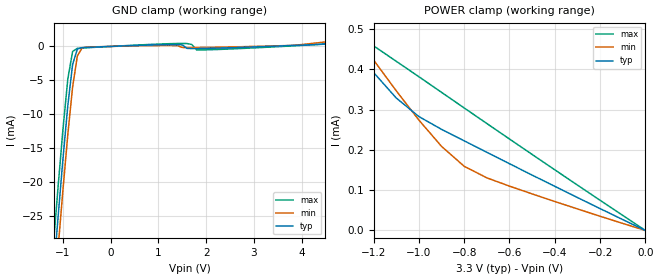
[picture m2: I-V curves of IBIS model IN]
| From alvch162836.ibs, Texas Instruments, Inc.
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|   Model ALVCH162836_IN
[Model]   IN
Model_type   Input
Polarity   Non-Inverting
Vinl = 0.8V
Vinh = 2.0V
|Variable   typ   min   max
C_comp   6pF   NA   NA
[Voltage Range]   3.3   3.0   3.6
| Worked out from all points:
|   GND clamp passes 1 mA (typ) near -0.73 V on its own axis
|   POWER clamp passes 1 mA (typ) near -1.97 V on its own axis
[POWER_Clamp]   | Note: Vtable = Vcc - Voutput
|   Voltage   I(typ)   I(min)   I(max)
-3.3V     2.121mA    2.168mA    2.076mA
-1.4V     540.7uA    581.6uA    541.7uA
-1.3V     464.2uA    501.6uA    497.2uA
-1.2V     392uA      423uA      458.1uA
-1.1V     328.8uA    346.6uA    419.8uA
-1V       282.6uA    273.9uA    381.5uA
-900mV    250.9uA    208.7uA    342.7uA
-800mV    222.4uA    159.2uA    304uA
-700mV    193.9uA    130.6uA    265.4uA
-600mV    165.6uA    110uA      226.9uA
-300mV    81.7uA     53.43uA    112.6uA
0V        1.064nA    1.048nA    1.063nA
[GND_Clamp]
|   Voltage   I(typ)   I(min)   I(max)
-3.3V     -228.9mA   -233.1mA   -224.8mA
-1.2V     -33.4mA    -38.07mA   -28.95mA
-1.1V     -24.73mA   -29.35mA   -20.28mA
-1V       -16.38mA   -20.91mA   -12.02mA
-900mV    -8.673mA   -12.94mA   -4.776mA
-800mV    -2.646mA   -5.969mA   -744.8uA
-700mV    -380.8uA   -1.394mA   -282.9uA
-600mV    -177.8uA   -207.9uA   -234.2uA
-500mV    -142.4uA   -98.01uA   -194.6uA
1.4V      255.6uA    108.4uA    429uA
3.8V      137.4uA    159.2uA    74.84uA
6.6V      2.121mA    2.422mA    1.823mA
